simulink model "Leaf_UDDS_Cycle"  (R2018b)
settings: Solver=VariableStepAuto  StartTime=0.0  StopTime=1369  FixedStep=1e-3  RelTol=1e-3
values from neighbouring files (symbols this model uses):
  B = 0    [Leaf_Initialization.m]    (also in PMSM_EV_init_v2.m; Tesla_Initialization.m)
  J = 0.3    [Leaf_Initialization.m]    (also in PMSM_EV_init_v2.m; Tesla_Initialization.m)
  Leaf_id_axis = [-2.296328E+02	-2.041181E+02	-1.786033E+02	-1.530886E+02	-1.275738E+02	-1.020590E+02	-7.654428E+01	-5.102952E+01	-2.551476E+01	+0.000000E+00]    [Leaf_Initialization.m]    (also in Leaf_Param.m)
  Leaf_iq_axis = [+0.000000E+00	+2.551476E+01	+5.102952E+01	+7.654428E+01	+1.020590E+02	+1.275738E+02	+1.530886E+02	+1.786033E+02	+2.041181E+02	+2.296328E+02]    [Leaf_Initialization.m]    (also in Leaf_Param.m)
  Leaf_Ld = [+4.562516E-04	+4.676675E-04	+4.893199E-04	+5.037353E-04	+5.104223E-04	+5.166612E-04	+5.237499E-04	+5.295159E-04	+5.345150E-04	+5.371060E-04    [Leaf_Initialization.m]    (also in Leaf_Param.m)
  Leaf_Lq = [+1.028048E-03	+1.047482E-03	+1.072792E-03	+1.100303E-03	+1.125549E-03	+1.152180E-03	+1.181188E-03	+1.211466E-03	+1.243133E-03	+1.273628E-03    [Leaf_Initialization.m]    (also in Leaf_Param.m)
  Leaf_omega_axis = [+0.000000E+00	+3.935365E+01	+7.870730E+01	+1.180610E+02	+1.574146E+02	+1.967683E+02	+2.361219E+02	+2.754756E+02	+3.857216E+02	+4.959676E+02	+6.062136E+02	+7.164596E+02	+8.267056E+02	+9.369516E+02	+1.047198E+03]    [Leaf_Initialization.m]    (also in Leaf_Param.m)
  Leaf_phid = [-4.199708E-02	-2.553401E-02	-8.247090E-03	+9.778563E-03	+2.810579E-02	+4.661402E-02	+6.539149E-02	+8.441129E-02	+1.036049E-01	+1.229854E-01    [Leaf_Initialization.m]    (also in Leaf_Param.m)
  Leaf_phiq = [-1.952292E-05	-3.396145E-06	+2.962394E-07	-2.077424E-05	-3.654397E-05	-1.649631E-05	+3.339687E-05	+4.306712E-05	+9.669480E-06	-2.373166E-05    [Leaf_Initialization.m]    (also in Leaf_Param.m)
  Leaf_torque_axis = [+0.000000E+00	+1.167089E+01	+2.334179E+01	+3.501268E+01	+4.668357E+01	+5.835446E+01	+7.002536E+01	+7.910792E+01	+9.076234E+01	+1.063042E+02	+1.281510E+02	+1.612785E+02	+2.121831E+02	+2.805757E+02]    [Leaf_Initialization.m]    (also in Leaf_Param.m)
  P = 8    [Leaf_Initialization.m]    (also in PMSM_EV_init_v2.m; Iqbal Husain - Example12_1.m = V.*I; Tesla_Initialization.m)
  Rs = 0.046    [Leaf_Initialization.m]    (also in PMSM_EV_init_v2.m; Tesla_Initialization.m)
undefined symbols (not defined in the file or in its folder): A1, B1370, HEV_Param
libraries: fl_lib x18, nesl_utility x9, sdl_lib x4

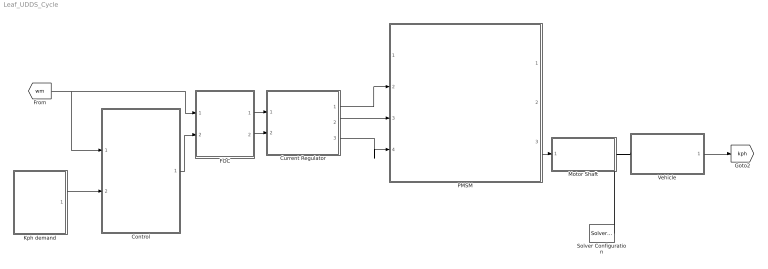
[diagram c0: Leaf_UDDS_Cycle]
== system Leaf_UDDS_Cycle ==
  Control : Subsystem
  Current Regulator : Subsystem
  FOC : Subsystem
  Kph demand : Subsystem
  Motor Shaft : Subsystem
  PMSM : Subsystem
  Solver Configuration : nesl_utility/Solver Configuration  PhysicalDomain=network_engine_domain  SubClassName=solver  LeftPortType=input  RightPortType=generic  Tones=[]  Harmonics=[]  SimulateNoise=off  Profile=off  UseLocalSampling=off  EnableSwitchedLinearOptims=on  FrequencyDomain=off  UseCCode=off  RelTol=0.001  AbsTol=1e-06  MinStep=1e-09  ToWorkspace=off  RevertToSquareIcSolve=off  NumHomotopyIterations=100  PhasorMode=off  PhasorModeNumHarmonics=1  DoDC=off  ResidualTolerance=1e-09  UseLocalSolver=off  LocalSolverChoice=NE_BACKWARD_EULER_ADVANCER  LocalSolverSampleTime=0.001  DoFixedCost=off  MaxNonlinIter=3  MaxModeIter=2  LinearAlgebra=auto  EquationFormulation=NE_TIME_EF  DelaysMemoryBudget=1024  AutomaticFiltering=on  FilteringTimeConstant=0.001  PartitionStorageMethod=AS_NEEDED  PartitionMemoryBudget=1024
  Vehicle : Subsystem
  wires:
  [wm] -> Control/1("rad/s "), FOC/1(Speed)
  FOC/2(Id_ref) -> Current Regulator/2(id_ref)
  PMSM/3(Torque (Nm)) -> Motor Shaft/1(In1)
  Current Regulator/2(Vb) -> PMSM/3(Vb)
  Control/1(Mot_TReq) -> FOC/2(Torque)
  Current Regulator/3(Vc) -> PMSM/4(Vc)
  Kph demand/1(Acc) -> Control/2(Acc)
  FOC/1(Iq_ref) -> Current Regulator/1(iq_ref)
  Current Regulator/1(Va) -> PMSM/2(Va)
  Vehicle/1(VehSpd) -> [kph]
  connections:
  Vehicle/LConn1 -- Solver Configuration/RConn1 -- Motor Shaft/RConn1

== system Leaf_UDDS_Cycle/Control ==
  "rad/s " : Inport
  Acc : Inport  Port=2
  Convert acceleration demand to motor speed demand. : Lookup  InputValues=[0 30]  Table=[0 10000]
  Gain : Gain  Gain=60/(2*pi)
  Motor Controller : Subsystem
  Mot_TReq : Outport
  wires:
  Motor Controller/1(M_Trq_Dem) -> Mot_TReq/1
  Convert acceleration demand to motor speed demand./1 -> Motor Controller/1(Mot_RPM_Dem)
  "rad/s "/1 -> Gain/1
  Acc/1 -> Convert acceleration demand to motor speed demand./1
  Gain/1 -> Motor Controller/2(Mot_RPM)

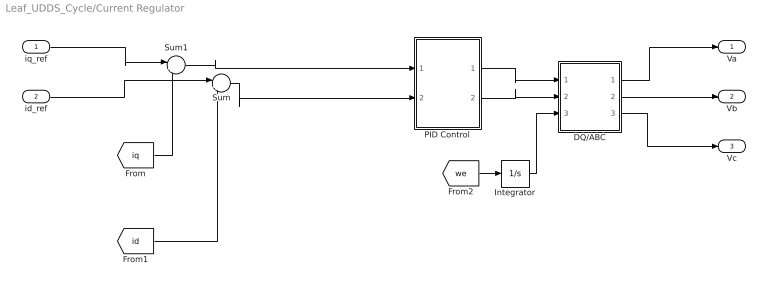
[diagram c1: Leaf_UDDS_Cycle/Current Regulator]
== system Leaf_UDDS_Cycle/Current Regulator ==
  iq_ref : Inport
  id_ref : Inport  Port=2
  DQ/ABC : Subsystem
  Integrator : Integrator
  PID Control : Subsystem
  Sum : Sum  Inputs=|+-
  Sum1 : Sum  Inputs=|+-
  Va : Outport
  Vb : Outport  Port=2
  Vc : Outport  Port=3
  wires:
  [iq] -> Sum1/2
  [id] -> Sum/2
  PID Control/1(Out1) -> DQ/ABC/1(Vq)
  Sum/1 -> PID Control/2(In3)
  PID Control/2(Out2) -> DQ/ABC/2(Vd)
  id_ref/1 -> Sum/1
  [we] -> Integrator/1
  iq_ref/1 -> Sum1/1
  Integrator/1 -> DQ/ABC/3(theta_rf)
  Sum1/1 -> PID Control/1(In1)
  DQ/ABC/3("Vc ") -> Vc/1
  DQ/ABC/1(Va) -> Va/1
  DQ/ABC/2("Vb ") -> Vb/1

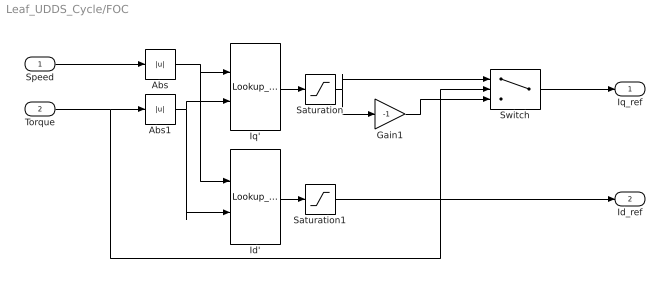
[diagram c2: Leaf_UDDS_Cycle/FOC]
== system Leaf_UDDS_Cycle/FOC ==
  Speed : Inport
  Torque : Inport  Port=2
  Abs : Abs
  Abs1 : Abs
  Gain1 : Gain  Gain=-1
  Id' : Lookup_n-D  BreakpointsForDimension1=Leaf_omega_axis  BreakpointsForDimension2=Leaf_torque_axis  Table=Leaf_Id'  InternalRulePriority=Speed  RndMeth=Simplest
  Iq' : Lookup_n-D  BreakpointsForDimension1=Leaf_omega_axis  BreakpointsForDimension2=Leaf_torque_axis  Table=Leaf_Iq'  InternalRulePriority=Speed  RndMeth=Simplest
  Saturation : Saturate  UpperLimit=300  LowerLimit=-300
  Saturation1 : Saturate  UpperLimit=300  LowerLimit=-300
  Switch : Switch  Criteria=u2 > Threshold
  Iq_ref : Outport
  Id_ref : Outport  Port=2
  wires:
  Abs/1 -> Id'/1, Iq'/1
  Abs1/1 -> Id'/2, Iq'/2
  Speed/1 -> Abs/1
  Id'/1 -> Saturation1/1
  Switch/1 -> Iq_ref/1
  Torque/1 -> Switch/2, Abs1/1
  Gain1/1 -> Switch/3
  Saturation/1 -> Switch/1, Gain1/1
  Saturation1/1 -> Id_ref/1
  Iq'/1 -> Saturation/1

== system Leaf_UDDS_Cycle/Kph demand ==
  From Spreadsheet3 : FromSpreadsheet  FileName=LA4_Cycle.xlsx  Range=A1:B1370  ExtrapolationBeforeFirstDataPoint=Hold first value
  Gain : Gain  Gain=1.6
  Vehicle Speed Controller : Subsystem
  Acc : Outport
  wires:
  From Spreadsheet3/1 -> Gain/1
  [kph] -> Vehicle Speed Controller/2(Veh Spd)
  Gain/1 -> Vehicle Speed Controller/1(Ref Spd)
  Vehicle Speed Controller/1(Acc) -> Acc/1

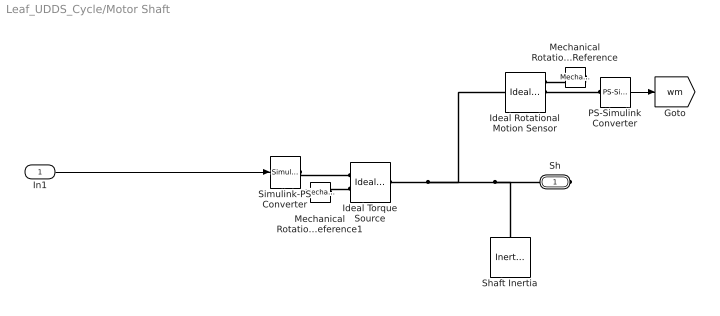
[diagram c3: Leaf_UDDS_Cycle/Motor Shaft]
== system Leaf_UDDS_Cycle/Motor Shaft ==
  In1 : Inport
  Ideal Rotational Motion Sensor : fl_lib/Mechanical/Mechanical Sensors/Ideal Rotational Motion Sensor  offset=0 rad
  Ideal Torque Source : fl_lib/Mechanical/Mechanical Sources/Ideal Torque Source
  Mechanical Rotational Reference : fl_lib/Mechanical/Rotational Elements/Mechanical Rotational Reference
  Mechanical Rotational Reference1 : fl_lib/Mechanical/Rotational Elements/Mechanical Rotational Reference
  PS-Simulink Converter : nesl_utility/PS-Simulink Converter  PhysicalDomain=network_engine_domain  SubClassName=ps_output  LeftPortType=input  RightPortType=output  PseudoPeriodic=off  Frequencies=[]  Unit=rad/s  AffineConversion=off
  Shaft Inertia : fl_lib/Mechanical/Rotational Elements/Inertia  inertia=HEV_Param.Motor.Shaft_Inertia kg*m^2  w_specify=on  w_priority=High  w=0 rad/s  w_nominal_specify=off  w_nominal_unit=rad/s  w_nominal_value=1  t_specify=off  t_priority=High  t=0 N*m  t_nominal_specify=off  t_nominal_unit=N*m  t_nominal_value=1
  Simulink-PS Converter : nesl_utility/Simulink-PS Converter  PhysicalDomain=network_engine_domain  SubClassName=ps_input  LeftPortType=input  RightPortType=output  PseudoPeriodic=off  Frequencies=[]  NoiseDistribution=none  NoiseParameters=[]  Unit=1  AffineConversion=off  FilteringAndDerivatives=zero  SimscapeFilterOrder=1  InputFilterTimeConstant=.001  UdotUserProvided=0
  Sh : PMIOPort  Side=Right
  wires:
  In1/1 -> Simulink-PS Converter/1
  PS-Simulink Converter/1 -> [wm]
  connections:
  Mechanical Rotational Reference1/LConn1 -- Ideal Torque Source/RConn2
  Ideal Torque Source/LConn1 -- Ideal Rotational Motion Sensor/LConn1 -- Shaft Inertia/LConn1 -- Sh/RConn1
  Simulink-PS Converter/RConn1 -- Ideal Torque Source/RConn1
  Mechanical Rotational Reference/LConn1 -- Ideal Rotational Motion Sensor/RConn1
  PS-Simulink Converter/LConn1 -- Ideal Rotational Motion Sensor/RConn2

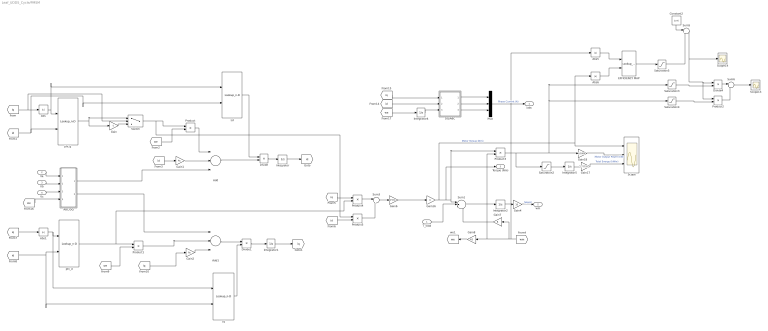
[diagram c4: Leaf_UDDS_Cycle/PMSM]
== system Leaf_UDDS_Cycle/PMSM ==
  T_load : Inport
  Va : Inport  Port=2
  Vb : Inport  Port=3
  Vc : Inport  Port=4
  ABC/DQ : Subsystem
  Abs{,1,5..6} (4 alike) : Abs
  Add : Sum  Inputs=+-+
  Add1 : Sum  Inputs=+--
  Constant2 : Constant  Value=1e-6
  DQ/ABC : Subsystem
  Divide : Product  Inputs=/*
  Divide1 : Product  Inputs=*/
  Divide4 : Product  Inputs=/*
  EFFICIENCY MAP : Lookup_n-D  BreakpointsForDimension1=Leaf_omega_axis  BreakpointsForDimension2=Leaf_torque_axis  Table=Leaf_Eff'  InternalRulePriority=Speed  RndMeth=Simplest
  Gain : Gain  Gain=-1
  Gain1 : Gain  Gain=Rs
  Gain16 : Gain
  Gain17 : Gain  Gain=2.77778e-7
  Gain18 : Gain  Gain=1/1000
  Gain2 : Gain  Gain=Rs
  Gain4 : Gain  Gain=1/J
  Gain6 : Gain  Gain=3*P/4
  Gain7 : Gain  Gain=B
  Gain8 : Gain  Gain=P/2
  Integrator{,1..2,4..5} (5 alike) : Integrator
  Ld : Lookup_n-D  BreakpointsForDimension1=Leaf_iq_axis  BreakpointsForDimension2=Leaf_id_axis  Table=Leaf_Ld  InternalRulePriority=Speed  RndMeth=Simplest
  Lq : Lookup_n-D  BreakpointsForDimension1=Leaf_iq_axis  BreakpointsForDimension2=Leaf_id_axis  Table=Leaf_Lq  InternalRulePriority=Speed  RndMeth=Simplest
  Mux : Mux  Inputs=3
  Product{,1..5} (6 alike) : Product
  Saturation2 : Saturate  UpperLimit=inf  LowerLimit=0
  Saturation3 : Saturate  UpperLimit=inf  LowerLimit=0
  Saturation4 : Saturate  UpperLimit=0  LowerLimit=-inf
  Saturation5 : Saturate  UpperLimit=inf  LowerLimit=0.1
  Scope : Scope  NumInputPorts=3
  Scope13 : Scope
  Scope14 : Scope
  Sum1 : Sum  Inputs=|+--
  Sum3 : Sum  Inputs=|+-
  Sum5 : Sum  Inputs=|++
  Sum6 : Sum  Inputs=|++
  Switch : Switch  Criteria=u2 > Threshold
  phi_d : Lookup_n-D  BreakpointsForDimension1=Leaf_iq_axis  BreakpointsForDimension2=Leaf_id_axis  Table=Leaf_phid  InternalRulePriority=Speed  RndMeth=Simplest
  phi_q : Lookup_n-D  BreakpointsForDimension1=Leaf_iq_axis  BreakpointsForDimension2=Leaf_id_axis  Table=Leaf_phiq  InternalRulePriority=Speed  RndMeth=Simplest
  iabc : Outport
  wm : Outport  Port=2
  Torque (Nm) : Outport  Port=3
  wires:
  [iq] -> Abs1/1
  Divide1/1 -> Integrator1/1
  [we] -> ABC/DQ/4(omega_rf)
  [id] -> Lq/2, phi_d/2
  [id] -> Ld/2, phi_q/2
  Vb/1 -> ABC/DQ/2(Vb)
  Integrator4/1 -> DQ/ABC/3(theta_rf)
  [we] -> Integrator4/1
  [iq] -> DQ/ABC/1(Iq)
  Abs/1 -> Ld/1, phi_q/1
  Divide/1 -> Integrator/1
  Add1/1 -> Divide1/1
  Gain1/1 -> Add/2
  [id] -> DQ/ABC/2(Id)
  Abs1/1 -> Lq/1, phi_d/1
  Integrator2/1 -> Gain4/1
  Ld/1 -> Divide/1
  [we] -> Product/2
  phi_q/1 -> Gain/1, Switch/1
  Product/1 -> Add/1
  Integrator1/1 -> [iq]
  T_load/1 -> Sum1/2
  [iq] -> Switch/2, Abs/1
  Add/1 -> Divide/2
  Sum1/1 -> Integrator2/1
  [we] -> Product1/2
  Va/1 -> ABC/DQ/1(Va)
  Integrator/1 -> [id]
  Gain/1 -> Switch/3
  Lq/1 -> Divide1/2
  Mux/1 -> iabc/1  "Phase Current (A)"
  Gain2/1 -> Add1/3
  DQ/ABC/2("Ib ") -> Mux/2
  DQ/ABC/3("Ic ") -> Mux/3
  Gain7/1 -> Sum1/3
  Gain8/1 -> [we]
  Product3/1 -> Saturation2/1, Saturation4/1, Saturation3/1, Gain18/1
  Integrator5/1 -> Gain17/1
  Gain17/1 -> Scope/3  "Total Energy (kWhr)"
  Gain18/1 -> Scope/2  "Motor Output Power (kW)"
  Saturation2/1 -> Integrator5/1
  Vc/1 -> ABC/DQ/3(Vc)
  ABC/DQ/2("q ") -> Add1/1
  [id] -> Gain1/1
  ABC/DQ/1(d) -> Add/3
  [iq] -> Gain2/1
  DQ/ABC/1(Ia) -> Mux/1
  phi_d/1 -> Product4/2, Product1/1
  Product1/1 -> Add1/2
  Switch/1 -> Product5/1, Product/1
  [wm] -> Abs5/1, Gain8/1, Product3/2, Gain7/1
  [iq] -> Product4/1
  Product4/1 -> Sum3/1
  [id] -> Product5/2
  Product5/1 -> Sum3/2
  Sum3/1 -> Gain6/1
  Gain6/1 -> Gain16/1
  EFFICIENCY MAP/1 -> Saturation5/1
  Saturation5/1 -> Sum5/2
  Abs5/1 -> EFFICIENCY MAP/1
  Divide4/1 -> Sum6/1
  Saturation3/1 -> Divide4/2
  Saturation4/1 -> Product2/2
  Constant2/1 -> Sum5/1
  Sum6/1 -> Scope13/1
  Gain16/1 -> Torque (Nm)/1, Product3/1, Sum1/1, Abs6/1, Scope/1  "Motor Torque (Nm)"
  Abs6/1 -> EFFICIENCY MAP/2
  Sum5/1 -> Scope14/1, Product2/1, Divide4/1
  Gain4/1 -> wm/1  "Speed"
  Product2/1 -> Sum6/2

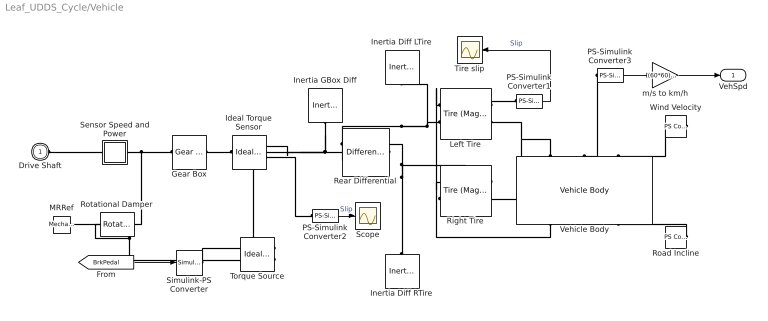
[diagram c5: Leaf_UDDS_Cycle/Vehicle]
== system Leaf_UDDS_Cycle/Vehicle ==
  Gear Box : fl_lib/Mechanical/Mechanisms/Gear Box  ratio=HEV_Param.Vehicle.Engine_Vehicle_Gear_Ratio  t_in_specify=off  t_in_priority=High  t_in=0 N*m  t_in_nominal_specify=off  t_in_nominal_unit=N*m  t_in_nominal_value=1  t_out_specify=off  t_out_priority=High  t_out=0 N*m  t_out_nominal_specify=off  t_out_nominal_unit=N*m  t_out_nominal_value=1
  Ideal Torque Sensor : fl_lib/Mechanical/Mechanical Sensors/Ideal Torque Sensor
  Inertia Diff LTire : fl_lib/Mechanical/Rotational Elements/Inertia  inertia=HEV_Param.Vehicle.Wheel_Inertia*2 kg*m^2  w_specify=on  w_priority=High  w=0 rad/s  w_nominal_specify=off  w_nominal_unit=rad/s  w_nominal_value=1  t_specify=off  t_priority=High  t=0 N*m  t_nominal_specify=off  t_nominal_unit=N*m  t_nominal_value=1
  Inertia Diff RTire : fl_lib/Mechanical/Rotational Elements/Inertia  inertia=HEV_Param.Vehicle.Wheel_Inertia*2 kg*m^2  w_specify=on  w_priority=High  w=0 rad/s  w_nominal_specify=off  w_nominal_unit=rad/s  w_nominal_value=1  t_specify=off  t_priority=High  t=0 N*m  t_nominal_specify=off  t_nominal_unit=N*m  t_nominal_value=1
  Inertia GBox Diff : fl_lib/Mechanical/Rotational Elements/Inertia  inertia=HEV_Param.Vehicle.Trans.Inertia kg*m^2  w_specify=on  w_priority=High  w=0 rad/s  w_nominal_specify=off  w_nominal_unit=rad/s  w_nominal_value=1  t_specify=off  t_priority=High  t=0 N*m  t_nominal_specify=off  t_nominal_unit=N*m  t_nominal_value=1
  Left Tire : sdl_lib/Tires & Vehicles/Tire (Magic Formula)  parameterization=1  F_z1=HEV_Param.Vehicle.Tire.Rated_Vertical_Load N  F_x1=HEV_Param.Vehicle.Tire.Rated_Peak_Long_Force N  kappa1=HEV_Param.Vehicle.Tire.Slip_At_Peak_Force  B_m=10  C_m=1.9  D_m=1  E_m=0.97  fz0=4e+3 N  p_Cx=1.685  p_Dx=[ 1.21 -0.037 ]  p_Ex=[ 0.344 0.095 -0.02 0 ]  p_Kx=[ 21.51 -0.163 0.245 ]  p_Hx=[ -0.002 0.002 ]  p_Vx=[ 0 0 ]  v_tr_thr=0.1 m/s  r_e=HEV_Param.Vehicle.Tire_Radius m  model_compliance=0  stiffness=1e+6 N/m  damping=1000 N/(m/s)  model_inertia=1  inertia=1e-2 kg*m^2  initial_velocity=0 rpm  model_resistance=1  resistance_model=1  coeff=0.015  p_tire=250e3 Pa  alpha=-0.003  beta=0.97  coeff_a=84e-4  coeff_b=6.2e-4 s/m  coeff_c=1.6e-4 s^2/m^2  v_thr=1e-3 m/s
  MRRef : fl_lib/Mechanical/Rotational Elements/Mechanical Rotational Reference
  PS-Simulink Converter1 : nesl_utility/PS-Simulink Converter  PhysicalDomain=network_engine_domain  SubClassName=ps_output  LeftPortType=input  RightPortType=output  PseudoPeriodic=off  Frequencies=[]  Unit=1  AffineConversion=off
  PS-Simulink Converter2 : nesl_utility/PS-Simulink Converter  PhysicalDomain=network_engine_domain  SubClassName=ps_output  LeftPortType=input  RightPortType=output  PseudoPeriodic=off  Frequencies=[]  Unit=1  AffineConversion=off
  PS-Simulink Converter3 : nesl_utility/PS-Simulink Converter  PhysicalDomain=network_engine_domain  SubClassName=ps_output  LeftPortType=input  RightPortType=output  PseudoPeriodic=off  Frequencies=[]  Unit=m/s  AffineConversion=off
  Rear Differential : sdl_lib/Gears/Differential  driveshaft_location=2  cd_ratio=1  friction_model=1  efficiency=[ 0.85 0.92 ]  mu_visc=[ 0 0 ] N*m/(rad/s)  pwr_thr=[ 0.001 0.001 ] W  carrier_inertia=0 kg*m^2  planet_inertia=0 kg*m^2  temperature_TLU=[ 280 300 320 ] K  efficiency_ss_TLU=[ 0.95 0.9 0.85 ]  efficiency_cd_TLU=[ 0.95 0.9 0.85 ]  thermal_mass=50 J/K  T_init=300 K
  Right Tire : sdl_lib/Tires & Vehicles/Tire (Magic Formula)  parameterization=1  F_z1=HEV_Param.Vehicle.Tire.Rated_Vertical_Load N  F_x1=HEV_Param.Vehicle.Tire.Rated_Peak_Long_Force N  kappa1=HEV_Param.Vehicle.Tire.Slip_At_Peak_Force  B_m=10  C_m=1.9  D_m=1  E_m=0.97  fz0=4e+3 N  p_Cx=1.685  p_Dx=[ 1.21 -0.037 ]  p_Ex=[ 0.344 0.095 -0.02 0 ]  p_Kx=[ 21.51 -0.163 0.245 ]  p_Hx=[ -0.002 0.002 ]  p_Vx=[ 0 0 ]  v_tr_thr=0.1 m/s  r_e=HEV_Param.Vehicle.Tire_Radius m  model_compliance=0  stiffness=1e+6 N/m  damping=1000 N/(m/s)  model_inertia=1  inertia=1e-2 kg*m^2  initial_velocity=0 rpm  model_resistance=1  resistance_model=1  coeff=0.015  p_tire=250e3 Pa  alpha=-0.003  beta=0.97  coeff_a=84e-4  coeff_b=6.2e-4 s/m  coeff_c=1.6e-4 s^2/m^2  v_thr=1e-3 m/s
  Road Incline : fl_lib/Physical Signals/Sources/PS Constant  constant=HEV_Param.Vehicle.Incline
  Rotational Damper : fl_lib/Mechanical/Rotational Elements/Rotational Damper  D=HEV_Param.Vehicle.Trans.Friction N*m/(rad/s)  w_specify=off  w_priority=High  w=0 rad/s  w_nominal_specify=off  w_nominal_unit=rad/s  w_nominal_value=1  t_specify=off  t_priority=High  t=0 N*m  t_nominal_specify=off  t_nominal_unit=N*m  t_nominal_value=1
  Scope : Scope
  Sensor Speed and Power : Subsystem
  Simulink-PS Converter : nesl_utility/Simulink-PS Converter  PhysicalDomain=network_engine_domain  SubClassName=ps_input  LeftPortType=input  RightPortType=output  PseudoPeriodic=off  Frequencies=[]  NoiseDistribution=none  NoiseParameters=[]  Unit=1  AffineConversion=off  FilteringAndDerivatives=zero  SimscapeFilterOrder=1  InputFilterTimeConstant=0.001  UdotUserProvided=1
  Tire slip : Scope
  Torque Source : fl_lib/Mechanical/Mechanical Sources/Ideal Torque Source
  Vehicle Body : sdl_lib/Tires & Vehicles/Vehicle Body  mass=HEV_Param.Vehicle.Mass kg  n_w=2  x_f=HEV_Param.Vehicle.Distance_CG_FrontAxle m  x_r=HEV_Param.Vehicle.Distance_CG_RearAxle m  y_c=HEV_Param.Vehicle.Distance_CG_Ground m  model_pitch=0  inertia=4000 kg*m^2  suspension_model=1  k_f=1e4 N/m  b_f=1e4 N/(m/s)  k_r=1e4 N/m  b_r=1e4 N/(m/s)  k_f_TLU=[-2000, -1000, 0, 1000, 2000] N  x_f_TLU=[-.4, -.2, 0, .2, .4] m  b_f_TLU=[-200, -100, 0, 100, 200] N  v_f_TLU=[-4, -2, 0, 2, 4] m/s  k_r_TLU=[-2000, -1000, 0, 1000, 2000] N  x_r_TLU=[-.4, -.2, 0, .2, .4] m  b_r_TLU=[-200, -100, 0, 100, 200] N  v_r_TLU=[-4, -2, 0, 2, 4] m/s  interp_method=simscape.enum.interpolation.linear  extrap_method=simscape.enum.extrapolation.linear  model_hardstop=0  upper_bound_f=.25 m  lower_bound_f=-.25 m  stop_k_f=1e6 N/m  stop_b_f=150 N/(m/s)  upper_bound_r=.25 m  lower_bound_r=-.25 m  stop_k_r=1e6 N/m  stop_b_r=150 N/(m/s)  initial_pitch=0 rad  initial_pitch_rate=0 rad/s  g=9.81 m/s^2  liftoff_warning=0  area=HEV_Param.Vehicle.Frontal_Area m^2  Cd=HEV_Param.Vehicle.Aero_Drag_Coeff  rho=1.18 kg/m^3  v_specify=on  v_priority=High  v=0 m/s  v_nominal_specify=off  v_nominal_unit=m/s  v_nominal_value=1
  Wind Velocity : fl_lib/Physical Signals/Sources/PS Constant  constant=0
  m/s to km/h : Gain  Gain=(60*60)/1000
  Drive Shaft : PMIOPort  Side=Left
  VehSpd : Outport
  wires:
  PS-Simulink Converter2/1 -> Scope/1  "Slip"
  PS-Simulink Converter3/1 -> m/s to km/h/1
  [BrkPedal] -> Simulink-PS Converter/1
  PS-Simulink Converter1/1 -> Tire slip/1  "Slip"
  m/s to km/h/1 -> VehSpd/1
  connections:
  Drive Shaft/RConn1 -- Sensor Speed and Power/LConn1
  Vehicle Body/LConn1 -- Right Tire/RConn2 -- Left Tire/RConn2
  Sensor Speed and Power/RConn1 -- Rotational Damper/LConn1 -- Gear Box/LConn1
  Torque Source/RConn2 -- Rotational Damper/RConn1 -- MRRef/LConn1
  Road Incline/RConn1 -- Vehicle Body/RConn3
  Inertia GBox Diff/LConn1 -- Rear Differential/LConn1 -- Torque Source/LConn1 -- Ideal Torque Sensor/RConn1
  Left Tire/RConn1 -- PS-Simulink Converter1/LConn1
  Wind Velocity/RConn1 -- Vehicle Body/LConn3
  Simulink-PS Converter/RConn1 -- Torque Source/RConn1
  PS-Simulink Converter2/LConn1 -- Ideal Torque Sensor/RConn2
  PS-Simulink Converter3/LConn1 -- Vehicle Body/LConn2
  Ideal Torque Sensor/LConn1 -- Gear Box/RConn1
  Vehicle Body/RConn1 -- Right Tire/LConn1 -- Left Tire/LConn1
  Left Tire/LConn2 -- Rear Differential/RConn2 -- Inertia Diff LTire/LConn1
  Rear Differential/RConn1 -- Right Tire/LConn2 -- Inertia Diff RTire/LConn1

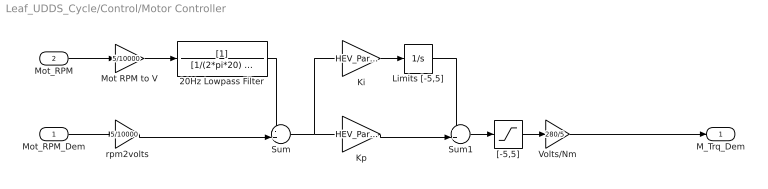
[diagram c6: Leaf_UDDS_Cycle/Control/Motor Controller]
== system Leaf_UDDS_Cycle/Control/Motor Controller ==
  Mot_RPM_Dem : Inport
  Mot_RPM : Inport  Port=2
  20Hz Lowpass Filter : TransferFcn  Denominator=[1/(2*pi*20) 1]
  Ki : Gain  Gain=HEV_Param.Control.Mot.Ki
  Kp : Gain  Gain=HEV_Param.Control.Mot.Kp
  Limits [-5,5] : Integrator  LimitOutput=on  UpperSaturationLimit=5  LowerSaturationLimit=-5
  Mot RPM to V : Gain  Gain=5/10000
  Sum : Sum  Inputs=-+|
  Sum1 : Sum  Inputs=++|
  Volts/Nm : Gain  Gain=280/5
  "[-5,5]" : Saturate  UpperLimit=5  LowerLimit=-5
  rpm2volts : Gain  Gain=5/10000
  M_Trq_Dem : Outport
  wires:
  "[-5,5]"/1 -> Volts/Nm/1
  Mot_RPM/1 -> Mot RPM to V/1
  Sum1/1 -> "[-5,5]"/1
  Sum/1 -> Ki/1, Kp/1
  Ki/1 -> Limits [-5,5]/1
  Kp/1 -> Sum1/2
  Limits [-5,5]/1 -> Sum1/1
  20Hz Lowpass Filter/1 -> Sum/1
  rpm2volts/1 -> Sum/2
  Mot RPM to V/1 -> 20Hz Lowpass Filter/1
  Mot_RPM_Dem/1 -> rpm2volts/1
  Volts/Nm/1 -> M_Trq_Dem/1

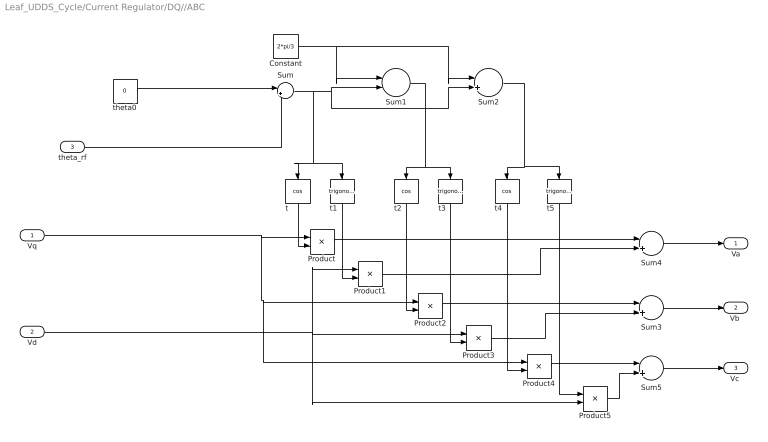
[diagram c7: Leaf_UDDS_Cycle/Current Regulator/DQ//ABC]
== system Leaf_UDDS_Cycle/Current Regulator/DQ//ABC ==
  Vq : Inport
  Vd : Inport  Port=2
  theta_rf : Inport  Port=3
  Constant : Constant  Value=2*pi/3
  Product{,1..5} (6 alike) : Product
  Sum{,2..5} (5 alike) : Sum  Inputs=|++
  Sum1 : Sum  Inputs=|-+
  t : Trigonometry  Operator=cos
  t1 : Trigonometry
  t2 : Trigonometry  Operator=cos
  t3 : Trigonometry
  t4 : Trigonometry  Operator=cos
  t5 : Trigonometry
  theta0 : Constant  Value=0
  Va : Outport
  "Vb " : Outport  Port=2
  "Vc " : Outport  Port=3
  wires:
  theta0/1 -> Sum/1
  Sum/1 -> t1/1, t/1, Sum2/2, Sum1/2
  Sum2/1 -> t5/1, t4/1
  Sum1/1 -> t2/1, t3/1
  t/1 -> Product/2
  Constant/1 -> Sum1/1, Sum2/1
  Product3/1 -> Sum3/2
  t1/1 -> Product1/2
  t3/1 -> Product3/2
  t2/1 -> Product2/2
  Sum4/1 -> Va/1
  Sum3/1 -> "Vb "/1
  theta_rf/1 -> Sum/2
  Vd/1 -> Product5/2, Product1/1, Product3/1
  Product/1 -> Sum4/1
  Product1/1 -> Sum4/2
  Product2/1 -> Sum3/1
  Vq/1 -> Product4/1, Product2/1, Product/1
  t4/1 -> Product4/2
  t5/1 -> Product5/1
  Product4/1 -> Sum5/1
  Product5/1 -> Sum5/2
  Sum5/1 -> "Vc "/1

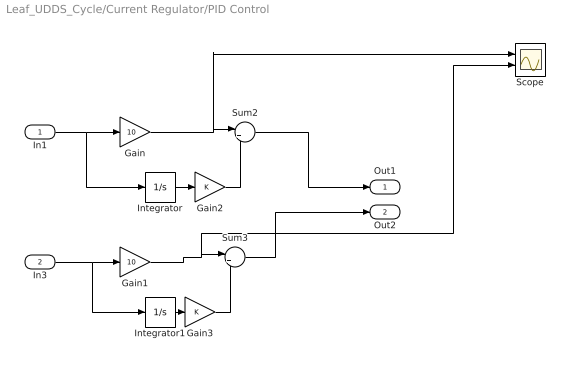
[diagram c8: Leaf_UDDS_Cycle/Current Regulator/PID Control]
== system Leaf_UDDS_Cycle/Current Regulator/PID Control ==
  In1 : Inport
  In3 : Inport  Port=2
  Gain : Gain  Gain=10
  Gain1 : Gain  Gain=10
  Gain2 : Gain
  Gain3 : Gain
  Integrator : Integrator
  Integrator1 : Integrator
  Scope : Scope  NumInputPorts=2
  Sum2 : Sum  Inputs=|++
  Sum3 : Sum  Inputs=|++
  Out1 : Outport
  Out2 : Outport  Port=2
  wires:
  Integrator1/1 -> Gain3/1
  Gain1/1 -> Scope/2, Sum3/1
  Gain2/1 -> Sum2/2
  Gain/1 -> Scope/1, Sum2/1
  In1/1 -> Integrator/1, Gain/1
  Sum2/1 -> Out1/1
  In3/1 -> Integrator1/1, Gain1/1
  Integrator/1 -> Gain2/1
  Gain3/1 -> Sum3/2
  Sum3/1 -> Out2/1

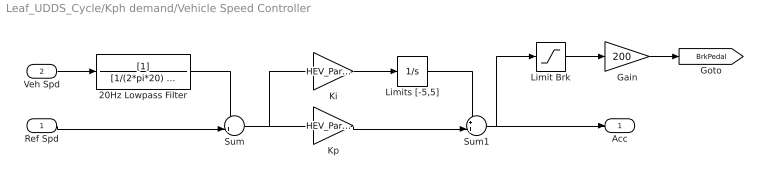
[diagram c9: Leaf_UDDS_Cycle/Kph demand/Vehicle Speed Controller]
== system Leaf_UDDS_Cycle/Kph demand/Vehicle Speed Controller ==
  Ref Spd : Inport
  Veh Spd : Inport  Port=2
  20Hz Lowpass Filter : TransferFcn  Denominator=[1/(2*pi*20) 1]
  Gain : Gain  Gain=200
  Ki : Gain  Gain=HEV_Param.Control.Veh_Spd.Ki
  Kp : Gain  Gain=HEV_Param.Control.Veh_Spd.Kp
  Limit Brk : Saturate  UpperLimit=0  LowerLimit=-inf
  Limits [-5,5] : Integrator  LimitOutput=on  UpperSaturationLimit=8  LowerSaturationLimit=-8
  Sum : Sum  Inputs=-+|
  Sum1 : Sum  Inputs=++|
  Acc : Outport
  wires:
  Ref Spd/1 -> Sum/2
  Veh Spd/1 -> 20Hz Lowpass Filter/1
  Sum/1 -> Ki/1, Kp/1
  Ki/1 -> Limits [-5,5]/1
  Kp/1 -> Sum1/2
  Limits [-5,5]/1 -> Sum1/1
  20Hz Lowpass Filter/1 -> Sum/1
  Limit Brk/1 -> Gain/1
  Gain/1 -> [BrkPedal]
  Sum1/1 -> Acc/1, Limit Brk/1

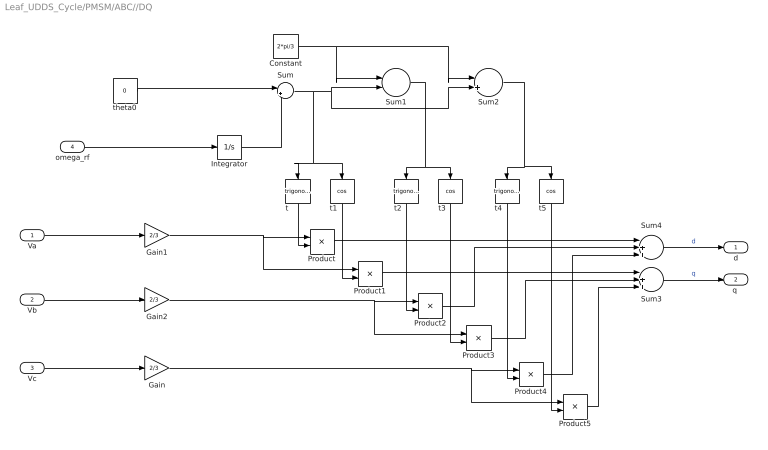
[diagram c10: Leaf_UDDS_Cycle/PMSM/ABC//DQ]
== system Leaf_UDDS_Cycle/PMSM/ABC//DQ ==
  Va : Inport
  Vb : Inport  Port=2
  Vc : Inport  Port=3
  omega_rf : Inport  Port=4
  Constant : Constant  Value=2*pi/3
  Gain : Gain  Gain=2/3
  Gain1 : Gain  Gain=2/3
  Gain2 : Gain  Gain=2/3
  Integrator : Integrator
  Product{,1..5} (6 alike) : Product
  Sum : Sum  Inputs=|++
  Sum1 : Sum  Inputs=|-+
  Sum2 : Sum  Inputs=|++
  Sum3 : Sum  Inputs=|+++
  Sum4 : Sum  Inputs=|+++
  t : Trigonometry
  t1 : Trigonometry  Operator=cos
  t2 : Trigonometry
  t3 : Trigonometry  Operator=cos
  t4 : Trigonometry
  t5 : Trigonometry  Operator=cos
  theta0 : Constant  Value=0
  d : Outport
  "q " : Outport  Port=2
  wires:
  theta0/1 -> Sum/1
  Sum/1 -> t1/1, t/1, Sum2/2, Sum1/2
  Sum2/1 -> t5/1, t4/1
  Integrator/1 -> Sum/2
  t4/1 -> Product4/2
  Sum1/1 -> t2/1, t3/1
  Product/1 -> Sum4/1
  t/1 -> Product/2
  Va/1 -> Gain1/1
  Constant/1 -> Sum1/1, Sum2/1
  Vc/1 -> Gain/1
  Product3/1 -> Sum3/2
  Gain2/1 -> Product3/1, Product2/1
  t5/1 -> Product5/2
  t1/1 -> Product1/2
  Gain/1 -> Product5/1, Product4/1
  Product1/1 -> Sum3/1
  Gain1/1 -> Product1/1, Product/1
  Product5/1 -> Sum3/3
  Product2/1 -> Sum4/2
  Product4/1 -> Sum4/3
  Vb/1 -> Gain2/1
  t3/1 -> Product3/2
  t2/1 -> Product2/2
  Sum4/1 -> d/1  "d"
  Sum3/1 -> "q "/1  "q"
  omega_rf/1 -> Integrator/1

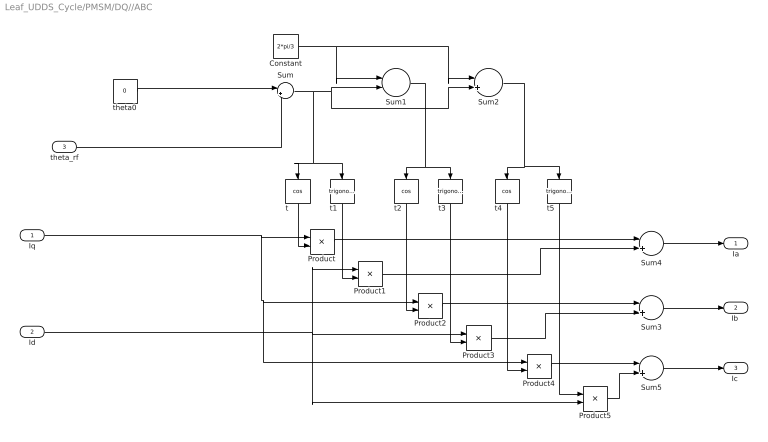
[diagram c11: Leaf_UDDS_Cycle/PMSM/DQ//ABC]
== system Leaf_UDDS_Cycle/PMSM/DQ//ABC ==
  Iq : Inport
  Id : Inport  Port=2
  theta_rf : Inport  Port=3
  Constant : Constant  Value=2*pi/3
  Product{,1..5} (6 alike) : Product
  Sum{,2..5} (5 alike) : Sum  Inputs=|++
  Sum1 : Sum  Inputs=|-+
  t : Trigonometry  Operator=cos
  t1 : Trigonometry
  t2 : Trigonometry  Operator=cos
  t3 : Trigonometry
  t4 : Trigonometry  Operator=cos
  t5 : Trigonometry
  theta0 : Constant  Value=0
  Ia : Outport
  "Ib " : Outport  Port=2
  "Ic " : Outport  Port=3
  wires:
  theta0/1 -> Sum/1
  Sum/1 -> t1/1, t/1, Sum2/2, Sum1/2
  Sum2/1 -> t5/1, t4/1
  Sum1/1 -> t2/1, t3/1
  t/1 -> Product/2
  Constant/1 -> Sum1/1, Sum2/1
  Product3/1 -> Sum3/2
  t1/1 -> Product1/2
  t3/1 -> Product3/2
  t2/1 -> Product2/2
  Sum4/1 -> Ia/1
  Sum3/1 -> "Ib "/1
  theta_rf/1 -> Sum/2
  Id/1 -> Product5/2, Product1/1, Product3/1
  Product/1 -> Sum4/1
  Product1/1 -> Sum4/2
  Product2/1 -> Sum3/1
  Iq/1 -> Product4/1, Product2/1, Product/1
  t4/1 -> Product4/2
  t5/1 -> Product5/1
  Product4/1 -> Sum5/1
  Product5/1 -> Sum5/2
  Sum5/1 -> "Ic "/1

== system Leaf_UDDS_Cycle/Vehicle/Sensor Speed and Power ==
  Ideal Rotational Motion Sensor : fl_lib/Mechanical/Mechanical Sensors/Ideal Rotational Motion Sensor  offset=0 rad
  Ideal Torque Sensor : fl_lib/Mechanical/Mechanical Sensors/Ideal Torque Sensor
  Mechanical Rotational Reference : fl_lib/Mechanical/Rotational Elements/Mechanical Rotational Reference
  PS-Simulink Converter : nesl_utility/PS-Simulink Converter  PhysicalDomain=network_engine_domain  SubClassName=ps_output  LeftPortType=input  RightPortType=output  PseudoPeriodic=off  Frequencies=[]  Unit=N*m  AffineConversion=off
  PS-Simulink Converter1 : nesl_utility/PS-Simulink Converter  PhysicalDomain=network_engine_domain  SubClassName=ps_output  LeftPortType=input  RightPortType=output  PseudoPeriodic=off  Frequencies=[]  Unit=rad/s  AffineConversion=off
  Product : Product
  W2kW : Gain  Gain=0.001
  B : PMIOPort  Side=Left
  F : PMIOPort  Port=2  Side=Right
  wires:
  W2kW/1 -> [Pm_vehicle]
  Product/1 -> W2kW/1
  PS-Simulink Converter/1 -> Product/1
  PS-Simulink Converter1/1 -> Product/2
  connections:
  Mechanical Rotational Reference/LConn1 -- Ideal Rotational Motion Sensor/RConn1
  Ideal Rotational Motion Sensor/LConn1 -- F/RConn1 -- Ideal Torque Sensor/RConn1
  B/RConn1 -- Ideal Torque Sensor/LConn1
  PS-Simulink Converter/LConn1 -- Ideal Torque Sensor/RConn2
  PS-Simulink Converter1/LConn1 -- Ideal Rotational Motion Sensor/RConn2
